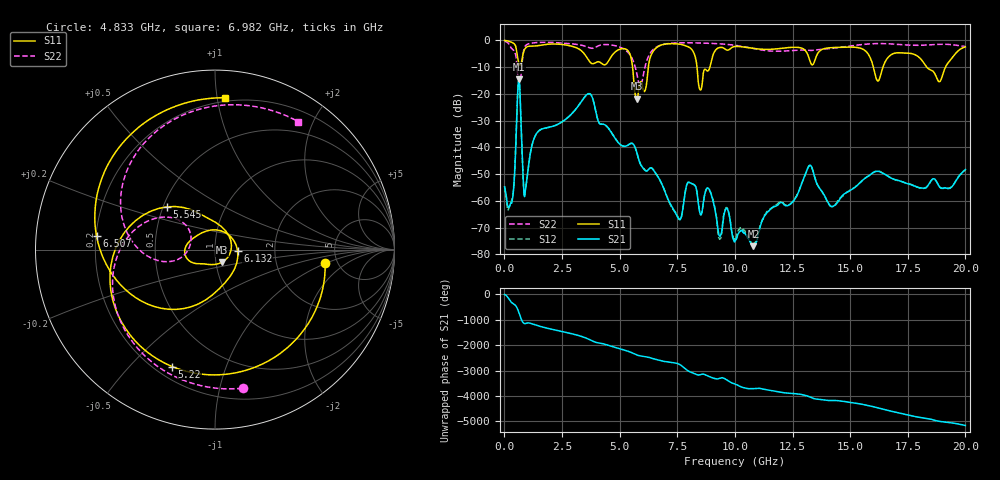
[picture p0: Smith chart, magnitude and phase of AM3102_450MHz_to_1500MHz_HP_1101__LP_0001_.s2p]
!Agilent Technologies,E8364B,MY43040894,A.07.50.67
!Agilent E8364B: A.07.50.67
!Date: Thursday, January 11, 2018 06:37:19
!Correction: S11(Full 2 Port(1,2))
!S21(Full 2 Port(1,2))
!S12(Full 2 Port(1,2))
!S22(Full 2 Port(1,2))
!S2P File: Measurements: S11, S21, S12, S22:
# Hz S  dB  R 50
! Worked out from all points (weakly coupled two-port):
!   1601 points, 10 MHz to 20 GHz, reference 50 ohm
!   highest |S21| = -14.66 dB at 634.7 MHz (marker M1); lowest = -77.0 dB at 10.8 GHz (marker M2)
!   lowest |S11| = -21.9 dB at 5.745 GHz (marker M3), VSWR 1.18, Z = 53.5 - j7.59 ohm
!   |S11| at or under -10 dB: 5.561 GHz to 6.244 GHz (683 MHz wide, 11.6 % of centre); 8.357 GHz to 8.916 GHz (558.7 MHz wide, 6.47 % of centre); 18.32 GHz to 19.14 GHz (819.2 MHz wide, 4.37 % of centre)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
!   |S22| runs from -17.0 to -0.4 dB; largest |S21 - S12| = 0.0023
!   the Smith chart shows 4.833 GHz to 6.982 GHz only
!   S11 on the Smith chart (normalised r, x): 4.833 GHz: 3.98, -0.97; 5.22 GHz: 0.26, -0.66; 5.545 GHz: 0.52, +0.29; 6.132 GHz: 1.29, -0.02; 6.507 GHz: 0.20, +0.05; 6.982 GHz: 0.17, +1.05
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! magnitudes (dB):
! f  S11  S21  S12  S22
! 10 MHz  -0.1  -54.8  -54.6  -0.4
! 334.8 MHz  -0.8  -60.1  -59.4  -3.2
! 634.7 MHz  -8.7  -14.7  -14.7  -15.4
! 909.5 MHz  -3.0  -56.1  -56.1  -2.1
! 1.409 GHz  -2.1  -34.7  -34.7  -0.8
! 3.346 GHz  -4.0  -22.8  -22.8  -1.8
! 4.833 GHz  -4.2  -37.0  -37.0  -2.1
! 5.22 GHz  -3.2  -39.6  -39.6  -3.5
! 5.545 GHz  -8.9  -38.5  -38.6  -6.8
! 5.745 GHz  -21.9  -41.9  -41.9  -12.5
! 6.132 GHz  -18.0  -48.8  -48.7  -8.9
! 6.507 GHz  -3.6  -49.0  -48.9  -3.1
! 6.682 GHz  -2.3  -51.3  -51.3  -2.2
! 6.982 GHz  -1.4  -56.9  -56.8  -1.4
! 8.493 GHz  -18.5  -64.8  -64.9  -1.0
! 10.01 GHz  -2.3  -75.1  -74.7  -1.9
! 10.8 GHz  -3.0  -77.0  -76.8  -3.1
! 13.34 GHz  -9.1  -47.6  -47.6  -3.8
! 14.22 GHz  -2.7  -62.2  -62.2  -3.0
! 16.68 GHz  -6.1  -51.0  -51.0  -1.3
! 18.86 GHz  -15.5  -54.6  -54.5  -1.5
! 20 GHz  -2.5  -48.3  -48.7  -2.3
